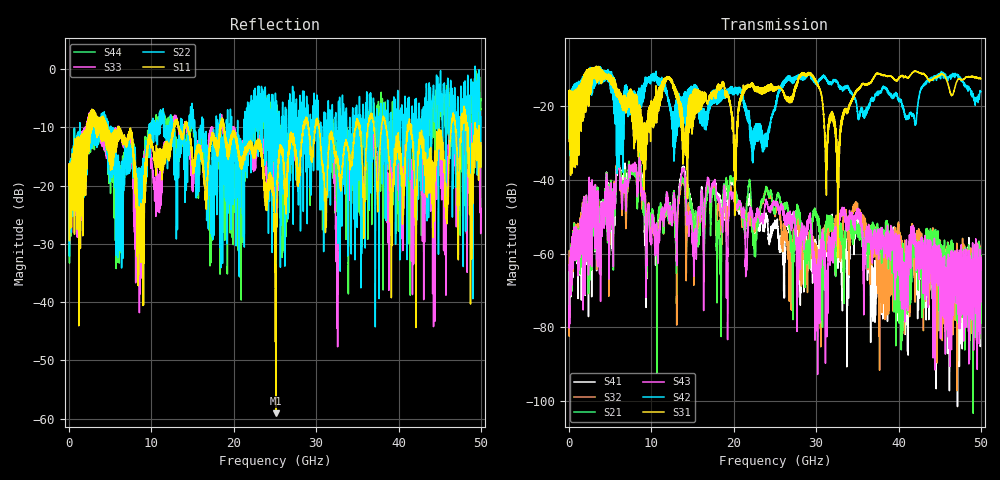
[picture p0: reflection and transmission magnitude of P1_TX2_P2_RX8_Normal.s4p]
!Keysight Technologies,N5225B,MY57041031,A.13.20.10
!Date: Friday, May 31, 2019 11:40:11
!Correction: S11(Full 4 Port(1,2,3,4))
!S12(Full 4 Port(1,2,3,4))
!S13(Full 4 Port(1,2,3,4))
!S14(Full 4 Port(1,2,3,4))
!S21(Full 4 Port(1,2,3,4))
!S22(Full 4 Port(1,2,3,4))
!S23(Full 4 Port(1,2,3,4))
!S24(Full 4 Port(1,2,3,4))
!S31(Full 4 Port(1,2,3,4))
!S32(Full 4 Port(1,2,3,4))
!S33(Full 4 Port(1,2,3,4))
!S34(Full 4 Port(1,2,3,4))
!S41(Full 4 Port(1,2,3,4))
!S42(Full 4 Port(1,2,3,4))
!S43(Full 4 Port(1,2,3,4))
!S44(Full 4 Port(1,2,3,4))
!S4P File: Measurements: <S11,S12,S13,S14>,
!<S21,S22,S23,S24>,
!<S31,S32,S33,S34>,
!<S41,S42,S43,S44>:
# Hz S  dB  R 50.0
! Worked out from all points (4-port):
!   5000 points, 10 MHz to 50 GHz, reference 50 ohm
!   strongest paths, dB at 10 MHz, 12.51 GHz, 25.01 GHz, 37.51 GHz, 50 GHz:
!     S31: -19.5, -13.0, -15.4, -11.1, -12.6
!     S42: -19.6, -21.8, -20.0, -16.4, -16.1
!     S43: -63.0, -52.5, -46.3, -53.6, -73.0
!     S21: -65.2, -48.4, -48.2, -55.9, -67.0
!     S32: -59.3, -51.3, -50.0, -67.7, -66.6
!     S41: -68.1, -50.3, -52.5, -58.8, -65.4
!   lowest |S11| = -59.1 dB at 25.1 GHz (marker M1), VSWR 1.00, Z = 49.9 + j0.0963 ohm
!   |S11| at or under -10 dB: 6.091 GHz to 12.71 GHz (6.615 GHz wide, 70.4 % of centre); 18.82 GHz to 28.43 GHz (9.603 GHz wide, 40.6 % of centre); 41.58 GHz to 46.39 GHz (4.81 GHz wide, 10.9 % of centre)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
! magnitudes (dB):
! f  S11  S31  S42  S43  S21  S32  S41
! 10 MHz  -19.8  -19.5  -19.6  -63.0  -65.2  -59.3  -68.1
! 5.97 GHz  -12.0  -16.7  -17.5  -34.0  -33.9  -33.5  -34.3
! 10.65 GHz  -13.7  -18.1  -12.3  -52.9  -92.4  -57.8  -55.9
! 25.1 GHz  -59.1  -15.1  -19.8  -46.3  -46.7  -48.2  -51.7
! 30.05 GHz  -9.3  -13.5  -13.8  -70.6  -49.1  -58.1  -61.6
! 32.64 GHz  -15.8  -37.7  -13.6  -52.6  -54.0  -54.2  -56.8
! 50 GHz  -12.6  -12.6  -16.1  -73.0  -67.0  -66.6  -65.4
